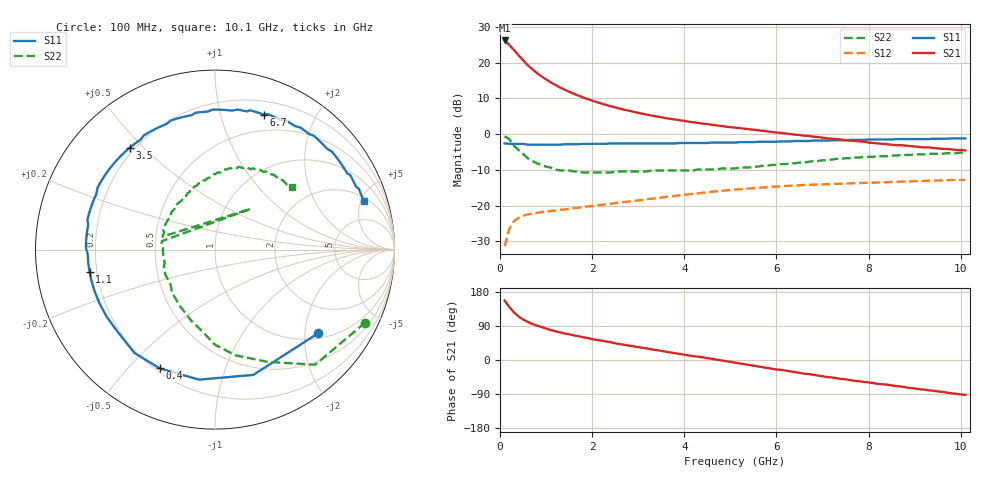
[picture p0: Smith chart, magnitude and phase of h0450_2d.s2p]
!HBFP-0450
!S and NOISE PARAMETERS at Vce=2V  Ic=10mA.  LAST UPDATED  09-04-98
# GHZ S MA R  50
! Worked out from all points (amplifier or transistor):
!   101 points, 100 MHz to 10.1 GHz, reference 50 ohm
!   highest |S21| = 26.2 dB at 100 MHz (marker M1)
!   |S21| within 3 dB of that: start of sweep to 324.6 MHz
!   unconditionally stable (mu >= 1): 2.702 GHz to end of sweep
!   at 1.7 GHz: K = 0.79, MSG = 15.7 dB, |S12| = -20.6 dB
!   at 5.1 GHz: K = 1.16, MAG = 6.2 dB, |S12| = -15.5 dB
!   at 10.1 GHz: K = 1.08, MAG = 2.4 dB, |S12| = -12.8 dB
!   lowest NFmin = 1.15 dB at 1.8 GHz
!   S11 on the Smith chart (normalised r, x): 100 MHz: 1.14, -2.34; 400 MHz: 0.22, -0.62; 1.1 GHz: 0.17, -0.08; 3.5 GHz: 0.18, +0.45; 6.7 GHz: 0.33, +1.38; 10.1 GHz: 2.38, +5.27
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0.1  0.74 -39.0  20.41 157.0  0.027 71.0  0.93 -26.0
0.2  0.73 -73.0  17.72 140.0  0.047 55.0  0.85 -49.0
0.3  0.73 -97.0  15.07 126.0  0.06 45.0  0.69 -65.0
0.4  0.73 -115.0  12.7 115.0  0.067 38.0  0.6 -79.0
0.5  0.73 -128.0  10.81 107.0  0.072 33.0  0.53 -90.0
0.6  0.71 -140.0  9.24 101.0  0.075 29.0  0.46 -99.0
0.7  0.71 -148.0  8.09 95.0  0.077 27.0  0.42 -108.0
0.8  0.71 -155.0  7.16 91.0  0.079 25.0  0.39 -115.0
0.9  0.71 -161.0  6.42 87.0  0.081 24.0  0.37 -122.0
1.1  0.71 -170.0  5.3 79.0  0.084 22.0  0.34 -135.0
1.4  0.72 179.0  4.19 70.0  0.088 21.0  0.31 -150.0
1.8  0.73 167.0  3.26 60.0  0.095 19.0  0.29 -165.0
2.1  0.73 159.0  2.8 53.0  0.1 19.0  0.29 -174.0
2.7  0.74 146.0  2.19 40.0  0.112 16.0  0.3 171.0
2.8  0.74 144.0  2.12 38.0  0.114 16.0  0.3 769.0
2.9  0.74 142.0  2.05 36.0  0.116 15.0  0.3 166.0
3.5  0.74 130.0  1.72 24.0  0.129 12.0  0.31 155.0
5.1  0.76 100.0  1.23 -7.0  0.167 -4.0  0.33 124.0
6.7  0.8 70.0  0.94 -37.0  0.195 -24.0  0.41 93.0
6.8  0.81 69.0  0.92 -39.0  0.196 -25.0  0.42 91.0
8.5  0.84 42.0  0.71 -67.0  0.214 -46.0  0.5 65.0
10.1  0.87 18.0  0.59 -92.0  0.229 -68.0  0.55 39.0
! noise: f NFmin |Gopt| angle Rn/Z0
1.8  1.15  0.46  177  0.05
2  1.21  0.48  -178  0.05
2.5  1.36  0.52  -163  0.06
3.5  1.63  0.62  -140  0.14
4  1.8  0.65  -127  0.25
5  2.09  0.7  -106  0.55
5.5  2.24  0.73  -95  0.81
7  2.67  0.77  -66  1.92
8  2.98  0.81  -49  2.94
10  3.56  0.83  -19  5.09
